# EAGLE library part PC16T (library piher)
POTENTIOMETER triple carbon potentiometer, 16 mm
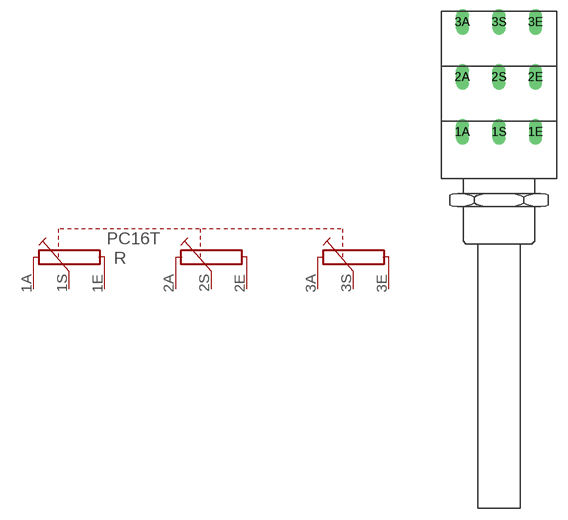
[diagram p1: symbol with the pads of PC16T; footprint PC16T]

Designator prefix R

## PC16T (OC_FARNELL: unknown; OC_NEWARK: unknown)  [PC16T]
1A  1A  pas
1E  1E  pas
1S  1S  pas
2A  2A  pas
2E  2E  pas
2S  2S  pas
3A  3A  pas
3E  3E  pas
3S  3S  pas

## Footprint PC16T (pad centres in mm)
POTENTIOMETER triple carbon potentiometer, 16 mm
drill 1.2 long: 1A -5,6.5; 1E 5,6.5; 1S 0,6.5; 2A -5,14; 2E 5,14; 2S 0,14; 3A -5,21.5; 3E 5,21.5; 3S 0,21.5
